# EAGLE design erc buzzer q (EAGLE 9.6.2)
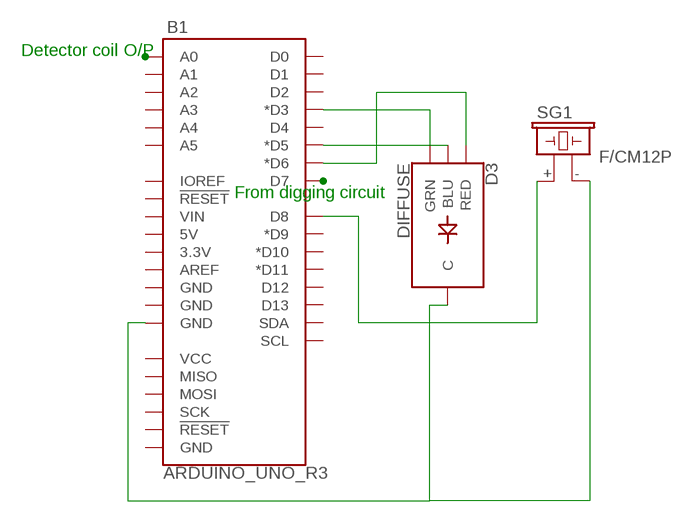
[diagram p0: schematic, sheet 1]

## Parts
B1  ARDUINO_UNO_R3  [ARDUINO_R3]
D3  DIFFUSE  LED-RGB-CCDIFFUSE  [LED-RGB-THRU]
SG1  F/CM12P  [F/CM12P]

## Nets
N$1: B1.D3(*D3) D3.3(GRN)
N$2: B1.GND@2(GND) D3.2(C) SG1.-
N$3: B1.D5(*D5) D3.4(BLU)
N$4: B1.D6(*D6) D3.1(RED)
N$5: B1.A0
N$6: B1.D8 SG1.+
N$7: B1.D7
Unconnected: B1.3.3V B1.5V B1.A1 B1.A2 B1.A3 B1.A4 B1.A5 B1.AREF B1.D0 B1.D1 B1.D2 B1.D4 B1.D9(*D9) B1.D10(*D10) B1.D11(*D11) B1.D12 B1.D13 B1.GND@1(GND) B1.GND@3(GND) B1.GND@4(GND) B1.IOREF B1.MISO B1.MOSI B1.RESET@1(!RESET!) B1.RESET@2(!RESET!) B1.SCK B1.SCL B1.SDA B1.VCC B1.VIN

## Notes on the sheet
- Detector coil O/P
- From digging circuit

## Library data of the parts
B1 = SparkFun-Boards:ARDUINO_UNO_R3: Arduino R3 Footprint with SPI header Arduino Uno R3 Compatible Footprint. Matches PCB size of the original board. SparkFun Products: SAMD21 Dev Breakout RedBoard R3 Stackable Headers
D3 = SparkFun-LED:LED-RGB-CC: LED-RGB Common Cathode Packages: LED RGB-THRU LED_PIRANHA_5MM SparkFun Products: RGB Diffused Common Cathode- Diffuse RGB Diffused Common Cathode - Clear LED-RGB 5mm Square (Piranha); PROD_ID: DIO-09434
SG1 = buzzer:F/CM12P: BUZZER; OC_FARNELL: unknown; OC_NEWARK: unknown

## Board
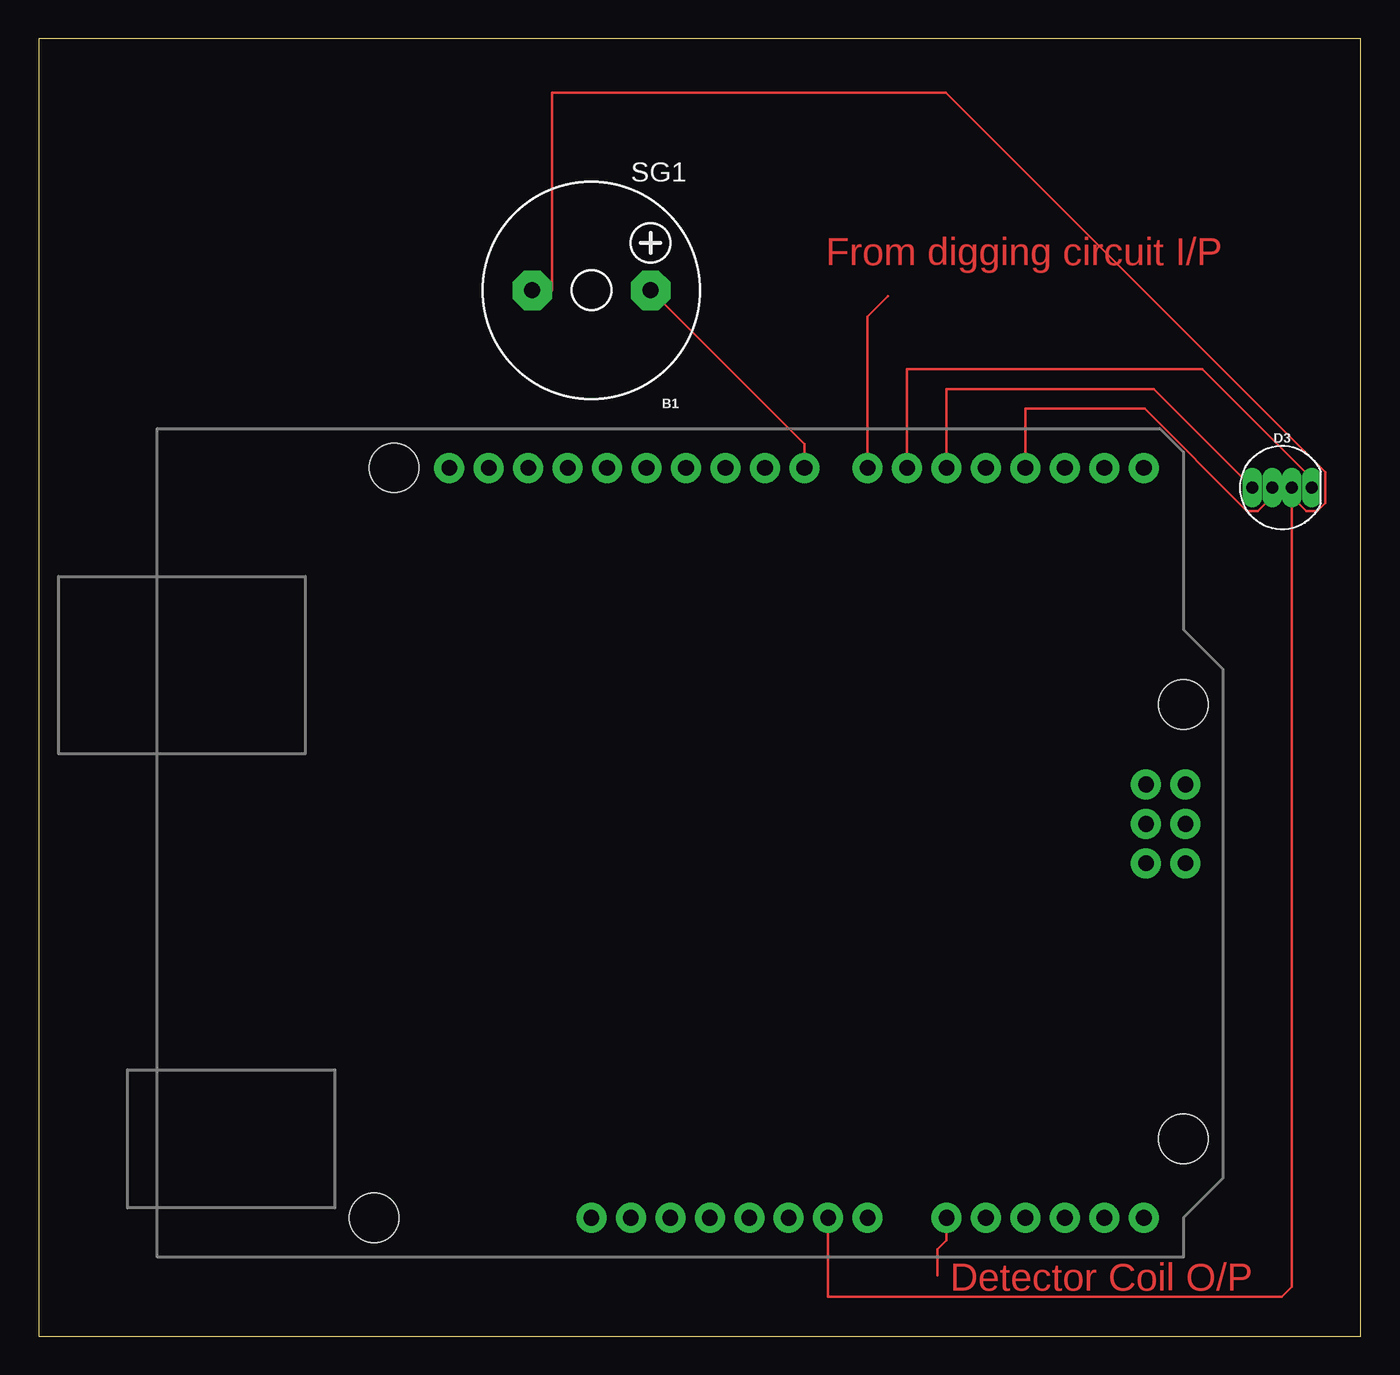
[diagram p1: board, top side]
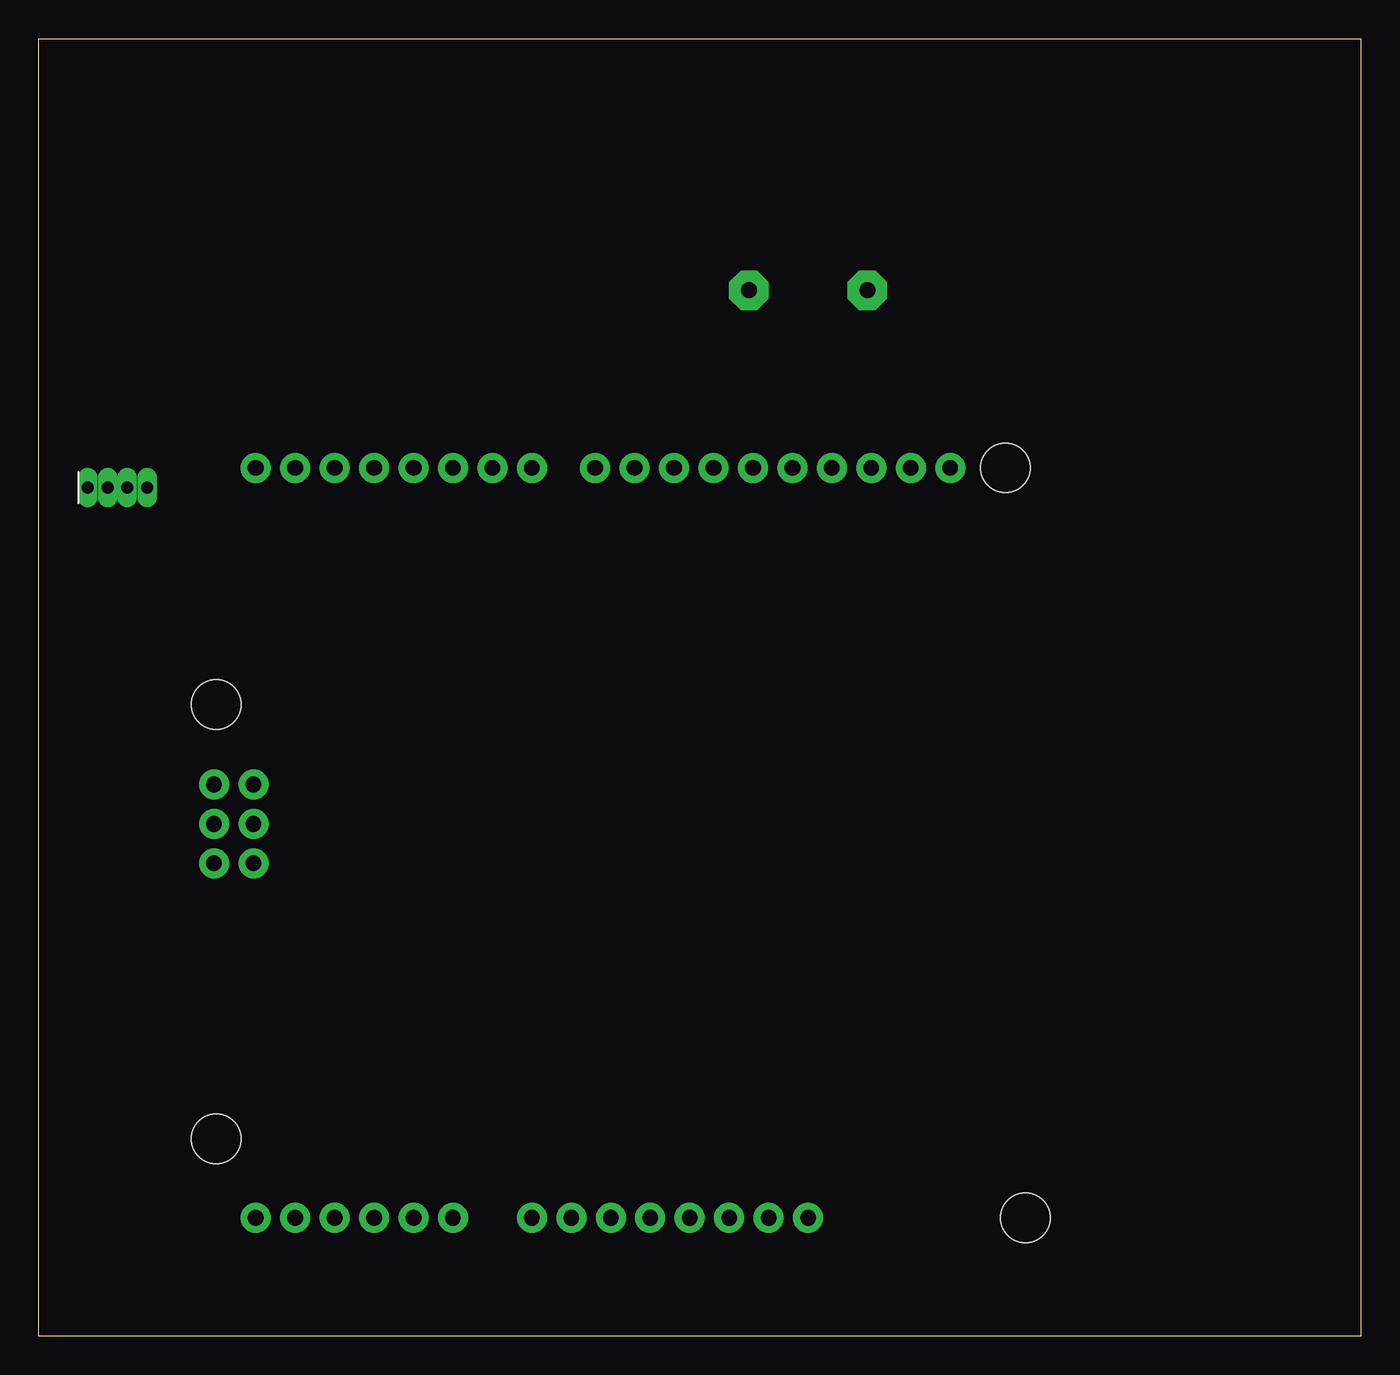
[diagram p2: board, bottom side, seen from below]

Size 85.07 x 83.49 mm. Coordinates in mm from the lower left corner, seen from the top.
Outline: 0,0 85.07,0 85.07,83.49 0,83.49 0,0
Copper layers (1*16): Top 0.035mm / dielectric 1.5mm / Bottom 0.035mm
Design rules "default": minimum track width 6mil, minimum drill 0.35mm, track to track 6mil, track to pad 6mil, pad to pad 6mil, via to via 6mil, smd to smd 6mil, copper to edge 40mil, drill to drill 6mil, minimum pad ring 10mil, minimum via ring 8mil, stop-mask expansion 4mil, vias tented up to drill 0mil, thermal gap 10mil

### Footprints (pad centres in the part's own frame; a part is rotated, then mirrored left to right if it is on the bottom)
ARDUINO_R3 = drill 1.016 pad 1.93: 3.3V 2.54,-24.13; 5V 5.08,-24.13; A0 17.78,-24.13; A1 20.32,-24.13; A2 22.86,-24.13; A3 25.4,-24.13; A4 27.94,-24.13; A5 30.48,-24.13; AREF -9.144,24.13; D0 30.48,24.13; D1 27.94,24.13; D2 25.4,24.13; D3 22.86,24.13; D4 20.32,24.13; D5 17.78,24.13; D6 15.24,24.13; D7 12.7,24.13; D8 8.636,24.13; D9 6.096,24.13; D10 3.556,24.13; D11 1.016,24.13; D12 -1.524,24.13; D13 -4.064,24.13; GND@1 7.62,-24.13; GND@2 10.16,-24.13; GND@3 -6.604,24.13; GND@4 33.16,-1.32; IOREF -2.54,-24.13; MISO 30.62,3.76; MOSI 33.16,1.22; NC -5.08,-24.13; RESET@1 0,-24.13; RESET@2 30.62,-1.32; SCK 30.62,1.22; SCL -14.224,24.13; SDA -11.684,24.13; VCC 33.16,3.76; VIN 12.7,-24.13 | hole 3.175: -17.78,24.13; 33.02,8.89; 33.02,-19.05; -19.05,-24.13
LED-RGB-THRU = drill 0.762 pad 0.889 long: 1 1.905,0; 2 0.635,0; 3 -0.635,0; 4 -1.905,0
F/CM12P = drill 1.016 pad 2.54 octagon: + 3.81,0; - -3.81,0

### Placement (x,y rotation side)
B1  40.64,31.75 0 top
D3  80.01,54.61 0 top
SG1  35.56,67.31 0 top

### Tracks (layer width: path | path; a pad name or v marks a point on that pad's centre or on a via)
N$1
  Top 0.152: B1.D3 63.5,59.69 71.17,59.69 77.75,53.11 78.46,53.11 78.97,53.62 78.97,54.2 D3.3
N$2
  Top 0.152: SG1.- 33.02,67.31 33.02,80.01 58.37,80.01 82.78,55.6 82.78,53.62 82.27,53.11 81.56,53.11 81.05,53.62 81.05,54.2 D3.2 80.65,3.18 80.01,2.54 50.8,2.54 B1.GND@2
N$3
  Top 0.152: D3.4 71.76,60.96 58.42,60.96 B1.D5
N$4
  Top 0.152: B1.D6 55.88,62.23 74.88,62.23 81.51,55.6 81.51,55.02 D3.1
N$5
  Top 0.152: 57.83,3.92 57.83,5.57 58.42,6.17 B1.A0
N$6
  Top 0.152: B1.D8 49.28,57.4 SG1.+
N$7
  Top 0.152: B1.D7 53.34,65.61 54.65,66.92

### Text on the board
Top: From digging circuit I/P | Detector Coil O/P

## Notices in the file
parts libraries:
SparkFun-Boards: Licensing: Creative Commons ShareAlike 4.0 International - https://creativecommons.org/licenses/by-sa/4.0
